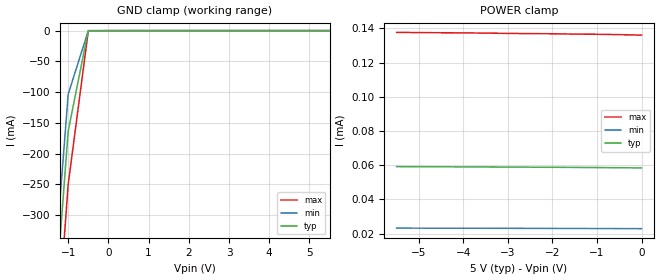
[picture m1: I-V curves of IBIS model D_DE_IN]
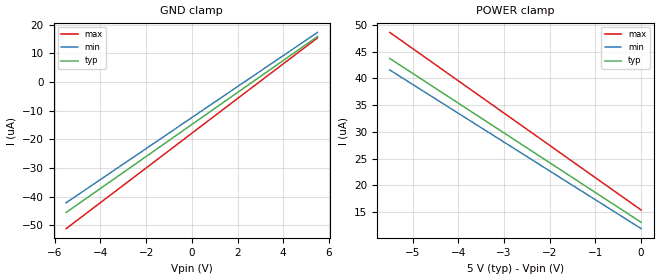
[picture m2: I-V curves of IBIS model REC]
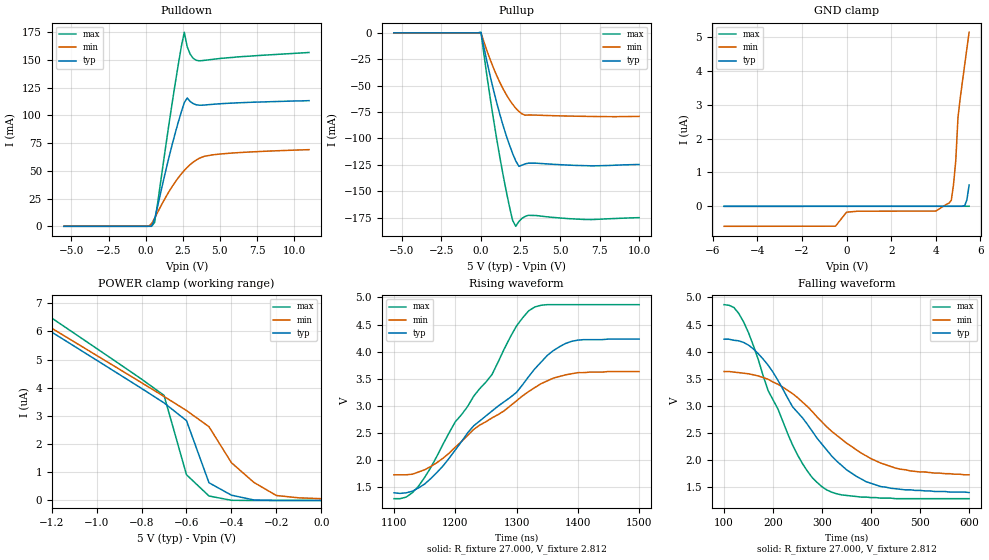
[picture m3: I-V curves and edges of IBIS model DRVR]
|   Texas Instruments Incorporated
|   Data Transmissions Products
|   IBIS Model for SN65HVD52
|   8D SOIC Package
[IBIS Ver]   3.2
[Comment char]   |_char
[File name]   hvd52.ibs
[File Rev]   1.0
[Date]   11Apr07
[Source]   File originated at Texas Instruments Incorporated.
   Data Transmission Products Group.
[Notes]
[Disclaimer]
(C) Copyright Texas Instruments Incorporated 2002
   All rights reserved
  Texas Instruments Incorporated hereby grants the user of this IBIS
model a non-exclusive, nontransferable license to use this IBIS model
under the following terms.  Before using this IBIS model, the user
should read this license.  If the user does not accept these terms,
the IBIS model should be returned to Texas Instruments within 30 days.
  The user is granted this license only to use the IBIS model and
is not granted rights to sell, load, rent, lease or license the IBIS
model in whole or in part, or in modified form to anyone other than
user.  User may modify the IBIS model to suit its specific applications
but rights to derivative works and such modifications shall belong to
Texas Instruments.
  This IBIS model is provided on an "AS IS" basis and Texas Instruments
makes absolutely no warranty with respect to the information contained
herein.  TEXAS INSTRUMENTS DISCLAIMS AND CUSTOMER WAIVES ALL WARRANTIES,
EXPRESS OR IMPLIED, INCLUDING WARRANTIES OF MERCHANTABILITY OR FITNESS
FOR A PARTICULAR PURPOSE. The entire risk as to quality and performance
is with the Customer. ACCORDINGLY, IN NO EVENT SHALL THE COMPANY BE LIABLE
FOR ANY DAMAGES, WHETHER IN CONTRACT OR TORT,INCLUDING ANY LOST PROFITS
OR OTHER INCIDENTAL, CONSEQUENTIAL, EXEMPLARY, OR PUNITIVE DAMAGES ARISING
OUT OF THE USE OR APPLICATION OF THE IBIS model provided in this package.
Further, Texas Instruments reserves the right to discontinue or make changes
without notice to any product herein to improve reliability, function, or
design. Texas Instruments does not convey any license under patent rights
or any other intellectual property rights, including those of third parties.
Contact Texas Instruments at ATTN:DATA TRANSMISSIONS
[Copyright]   Copyright 2002, Texas Instruments, All Rights Reserved
[Component]   HVD52D
[Manufacturer]  Texas Instruments Incorporated
[Package]
|   typ   min   max
R_pkg   0.071   0.050   0.091
L_pkg   2.203nH   1.540nH   2.930nH
C_pkg   0.465pF   0.385pF   0.609pF
[Pin]   signal_name   model_name   R_pin   L_pin   C_pin
1   VCC   POWER   0.091   2.615n   0.500p
2   R   RECEIVER_OUT   0.076   2.346n   0.483p
3   D   D_DE_IN   0.062   1.755n   0.395p
4   GND   GND   0.090   2.593n   0.498p
5   Y   DRVR   0.073   2.300n   0.480p
6   Z   DRVR   0.076   2.012n   0.407p
7   B   REC   0.050   1.540n   0.385p
8   A   REC   0.070   1.897n   0.412p
[Diff_pin]   inv_pin   vdiff   tdelay_typ   tdelay_min   tdelay_max
| The 'A' pin is Diff_pin and the 'B' pin is the inv_pin
5   6   0.200   0 0 0
7   8   0.200   0 0 0
| Models and submodels in the file (4): D_DE_IN (Input), REC (Input), DRVR (I/O), RECEIVER_OUT (3-state)
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|   Driver Input / Driver Enable / Model
[Model]   D_DE_IN
Model_type   Input
|Signals   D
Vinh = 2.0
Vinl = 0.8
|   typ   min   max
C_comp   23pF   19pF   27pF
|   typ   min   max
[Temperature Range]   27   -40   85
[Voltage range]   5.0V   4.5V   5.5V
[GND_clamp]
|   Voltage   I(typ)   I(min)   I(max)
-5.5V     -3.894A    -3.744A    -4.095A
-1.5V     -596.3mA   -523.6mA   -696.4mA
-1V       -163.5mA   -103.3mA   -250mA
-500mV    -18.38uA   -37.25uA   -400.5uA
5.5V      58.51uA    136uA      22.98uA
[Power_clamp]
| Note that the[POWER_clamp]voltage table is referenced to Vcc
| and is calculated using Vtable=Vcc - Vmeasured.
|   Voltage   I(typ)   I(min)   I(max)
-5.5V     59.15uA    23.21uA    137.6uA
-5V       59.11uA    23.19uA    137.5uA
-4.5V     59.06uA    23.17uA    137.4uA
-4V       59.01uA    23.15uA    137.3uA
-3.5V     58.95uA    23.12uA    137.2uA
-3V       58.9uA     23.1uA     137uA
-2.5V     58.83uA    23.07uA    136.9uA
-2V       58.77uA    23.04uA    136.8uA
-1.5V     58.69uA    23.01uA    136.6uA
-1V       58.61uA    22.98uA    136.5uA
-500mV    58.51uA    22.94uA    136.3uA
0V        58.4uA     22.9uA     136uA
|   Receiver Input / Model
[Model]   REC
Model_type   Input
|Signals   A,B
Vinh = 2.0
Vinl = 0.8
|   typ   min   max
C_comp   3.0pF   2.5pF   3.5pF
|   typ   min   max
[Temperature Range]   27   -40   85
[Voltage range]   5.0V   4.5V   5.5V
[GND_clamp]
|   Voltage   I(typ)   I(min)   I(max)
-5.5V     -45.49uA   -42.11uA   -51.13uA
-2V       -25.98uA   -23.22uA   -29.99uA
1.5V      -6.431uA   -4.293uA   -8.781uA
5.5V      15.87uA    17.3uA     15.38uA
[Power_clamp]
| Note that the[POWER_clamp]voltage table is referenced to Vcc
| and is calculated using Vtable=Vcc - Vmeasured.
|   Voltage   I(typ)   I(min)   I(max)
-5.5V     43.73uA    41.58uA    48.61uA
-5V       40.95uA    38.88uA    45.59uA
-4.5V     38.16uA    36.18uA    42.57uA
-4V       35.37uA    33.48uA    39.55uA
-3.5V     32.59uA    30.78uA    36.53uA
-3V       29.8uA     28.09uA    33.51uA
-2.5V     27.01uA    25.39uA    30.49uA
-2V       24.23uA    22.69uA    27.47uA
-1.5V     21.44uA    19.99uA    24.44uA
-1V       18.65uA    17.3uA     21.42uA
-500mV    15.87uA    14.6uA     18.4uA
0V        13.08uA    11.9uA     15.38uA
|   Driver Output / Receiver Input Model
[Model]   DRVR
Model_type   I/O
| Signals   Y,Z
Vinl = 0.9V
Vinh = 2.8V
Vmeas = 1.7V   |Reference voltage for timing measurements
Cref = 50pF   |Timing specification test load capacitance value
Rref = 54   |Note: 54 Ohm load; single-ended configuration
|   Timing specification test load voltage
| variable   typ   min   max
C_comp   28pF   24pF   32pF
|   typ   min   max
[Temperature Range]   25.0   -40   85
[Voltage range]   5.0V   4.5V   5.5V
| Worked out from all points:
|   slope of the pulldown table from 0 to 0.75 V, typ, clamps not added: 50.7 ohm
|   slope of the pullup table from 0 to 0.75 V, typ, clamps not added: 14.5 ohm
|   rising waveform, R_fixture 27.000, V_fixture 2.812: 20-80 % time 144ns typ, 130ns min, 118ns max; typ from 1.4 V to 4.23 V
|   falling waveform, R_fixture 27.000, V_fixture 2.812: 20-80 % time 135ns typ, 148ns min, 97.5ns max; typ from 4.23 V to 1.4 V
[Pulldown]
|   Voltage   I(typ)   I(min)   I(max)
-5.5V     -10.66pA   -1.61nA    -2.66pA
200mV     102.2nA    81.88uA    446.1pA
400mV     121.7uA    2.397mA    2.576uA
600mV     6.248mA    7.209mA    3.471mA
1.8V      74.35mA    36.14mA    112.4mA
2.4V      103mA      47.21mA    161.8mA
2.6V      111.4mA    50.31mA    174.8mA
2.8V      115.6mA    53.11mA    161.7mA
3V        112.4mA    55.6mA     155mA
3.6V      109.1mA    61.2mA     149.1mA
5.5V      110.8mA    65.68mA    151.8mA
11V       113.2mA    69.05mA    156.6mA
[Pullup]
|   Voltage   I(typ)   I(min)   I(max)
| Note that the[Pullup]voltage table is referenced to Vcc
| and is calculated using Vtable=Vcc - Vmeasured.
-5.5V     2.4uA      2.144uA    2.981uA
0V        269.5uA    177uA      535.4uA
600mV     -42.03mA   -26mA      -63.31mA
1.2V      -77.48mA   -47.12mA   -118.3mA
1.6V      -97.35mA   -58.48mA   -150.1mA
2V        -114.2mA   -67.65mA   -177.6mA
2.2V      -121.3mA   -71.41mA   -183.3mA
2.4V      -126.5mA   -74.49mA   -178.7mA
2.8V      -124.1mA   -78.04mA   -173.9mA
3V        -123.5mA   -77.81mA   -172.9mA
6.5V      -125.8mA   -79.1mA    -176.8mA
10V       -124.7mA   -79.14mA   -175.1mA
[GND_clamp]
|   Voltage  I(typ)   I(min)   I(max)
| Outputs in High Impedance (off)
-5.5V     -1.17nA    -592nA     -1.094nA
-500mV    -651.3pA   -589.2nA   -574.5pA
0V        -526.7pA   -174.9nA   -522.6pA
4V        256.2pA    -142.8nA   173.6pA
4.6V      361.5pA    94.35nA    277.1pA
4.7V      380.1pA    176.4nA    294pA
4.8V      394.4pA    641.3nA    311.8pA
4.9V      418.3pA    1.34uA     326.9pA
5V        446.8pA    2.618uA    343.7pA
5.3V      18.21nA    4.177uA    389pA
5.4V      188.2nA    4.662uA    400.6pA
5.5V      629.7nA    5.145uA    417.4pA
[POWER_clamp]
|   Voltage  I(typ)   I(min)   I(max)
| Note that the [POWER_clamp] voltage table is referenced to Vcc
| and is calculated using Vtable = Vcc - Vmeasured.
| Outputs in Tri-state.
-5.5V     27.39uA    26.86uA    29.68uA
-1.5V     7.468uA    7.559uA    8.092uA
-1.4V     6.97uA     7.077uA    7.552uA
-1.3V     6.472uA    6.594uA    7.012uA
-800mV    3.975uA    4.177uA    4.305uA
-700mV    3.462uA    3.69uA     3.728uA
-600mV    2.832uA    3.19uA     913.7nA
-500mV    629.7nA    2.618uA    159.9nA
-400mV    188.2nA    1.34uA     5.888nA
-300mV    18.21nA    641.3nA    839.3pA
-200mV    1.35nA     176.4nA    418.3pA
0V        446.8pA    64.16nA    417.4pA
[Ramp]
|   typ   min   max
dV/dt_r   1.68V/144ns   1.12V/130ns   2.13V/118ns
dV/dt_f   1.68V/145ns   1.08V/150ns   2.15V/114ns
R_load = 27ohm | Note: The measurement is on a single-ended configuration
|   with 54ohm line-to-line.
[Rising Waveform]
R_fixture = 27.000
V_fixture = 2.812
V_fixture_min = 2.663
V_fixture_max = 3.070
C_fixture = 0.000
L_fixture = 0.000
|  time   V(typ)   V(min)   V(max)
1.1us     1.395V     1.728V     1.287V
1.14us    1.486V     1.779V     1.518V
1.18us    1.891V     2.034V     2.292V
1.23us    2.631V     2.564V     3.177V
1.26us    2.905V     2.778V     3.579V
1.3us     3.249V     3.093V     4.474V
1.32us    3.543V     3.266V     4.755V
1.35us    3.928V     3.46V      4.867V
1.39us    4.191V     3.592V     4.867V
1.5us     4.232V     3.633V     4.867V
[Falling Waveform]
R_fixture = 27.000
V_fixture = 2.812
V_fixture_min = 2.663
V_fixture_max = 3.070
C_fixture = 0.000
L_fixture = 0.000
|  time   V(typ)   V(min)   V(max)
100ns     4.23V      3.633V     4.867V
130ns     4.2V       3.613V     4.706V
170ns     3.96V      3.551V     3.849V
190ns     3.75V      3.49V      3.28V
240ns     2.98V      3.224V     2.274V
270ns     2.66V      2.988V     1.796V
300ns     2.29V      2.701V     1.506V
350ns     1.82V      2.312V     1.347V
420ns     1.51V      1.943V     1.297V
600ns     1.4V       1.728V     1.287V
